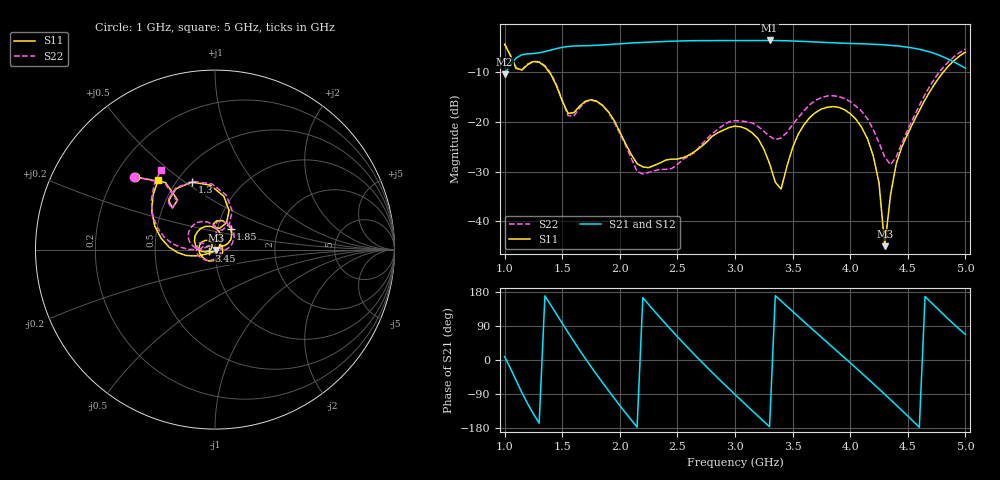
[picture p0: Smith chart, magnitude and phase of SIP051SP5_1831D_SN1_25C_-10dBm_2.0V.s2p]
# GHz  S  dB  R  50
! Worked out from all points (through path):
!   81 points, 1 GHz to 5 GHz, reference 50 ohm
!   highest |S21| = -3.65 dB at 3.3 GHz (marker M1); lowest = -10.4 dB at 1 GHz (marker M2)
!   lowest |S11| = -45.0 dB at 4.3 GHz (marker M3), VSWR 1.01, Z = 50.5 - j0.2 ohm
!   |S11| at or under -10 dB: 1.386 GHz to 4.809 GHz (3.423 GHz wide, 110 % of centre)
!   |S22| runs from -30.5 to -4.3 dB; largest |S21 - S12| = 0.0029
!   S11 on the Smith chart (normalised r, x): 1 GHz: 0.28, +0.36; 1.3 GHz: 0.60, +0.53; 1.85 GHz: 1.15, +0.28; 3.45 GHz: 0.93, -0.01; 5 GHz: 0.40, +0.41
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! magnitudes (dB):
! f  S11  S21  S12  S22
! 1 GHz  -4.4  -10.4  -10.4  -4.3
! 1.1 GHz  -9.2  -7.2  -7.2  -9.3
! 1.3 GHz  -8.0  -6.1  -6.1  -8.0
! 1.55 GHz  -18.3  -4.9  -4.9  -18.7
! 1.7 GHz  -15.9  -4.7  -4.7  -16.0
! 1.85 GHz  -16.7  -4.6  -4.6  -16.7
! 2.15 GHz  -28.4  -4.1  -4.1  -30.0
! 2.35 GHz  -28.3  -3.9  -3.9  -29.5
! 3 GHz  -20.9  -3.7  -3.7  -19.8
! 3.2 GHz  -23.4  -3.7  -3.7  -20.9
! 3.3 GHz  -28.4  -3.7  -3.7  -22.9
! 3.4 GHz  -33.5  -3.7  -3.7  -23.2
! 3.45 GHz  -29.0  -3.7  -3.7  -22.1
! 3.7 GHz  -18.1  -4.0  -4.0  -15.7
! 3.9 GHz  -17.1  -4.2  -4.2  -14.9
! 4.1 GHz  -21.1  -4.3  -4.3  -17.9
! 4.25 GHz  -32.3  -4.5  -4.5  -24.2
! 4.3 GHz  -45.0  -4.5  -4.5  -27.1
! 4.35 GHz  -34.7  -4.6  -4.6  -28.6
! 4.45 GHz  -25.0  -4.9  -4.9  -24.2
! 4.6 GHz  -17.8  -5.4  -5.4  -16.7
! 5 GHz  -6.0  -9.2  -9.3  -5.4
